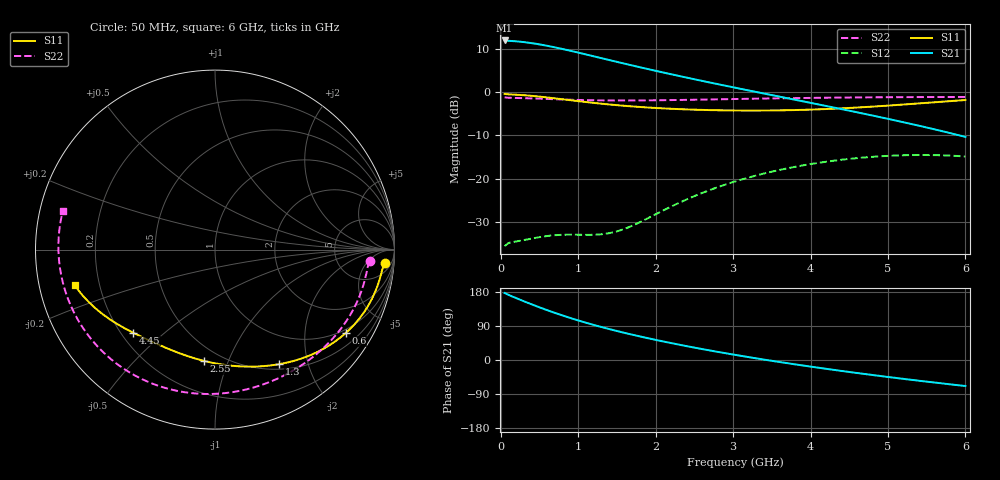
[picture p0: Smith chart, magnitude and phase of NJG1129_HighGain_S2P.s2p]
!S parameter
! Frequency  S11  S21  S12  S22
# HZ  S  DB R 50
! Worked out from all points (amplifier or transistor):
!   120 points, 50 MHz to 6 GHz, reference 50 ohm
!   highest |S21| = 11.9 dB at 50 MHz (marker M1)
!   |S21| within 3 dB of that: start of sweep to 1.047 GHz
!   unconditionally stable (mu >= 1): 116.3 MHz to 2.346 GHz
!   at 1.05 GHz: K = 1.47, MAG = 16.8 dB, |S12| = -33.0 dB
!   at 3.05 GHz: K = 0.66, MSG = 10.7 dB, |S12| = -20.5 dB
!   at 6 GHz: K = 0.66, MSG = 2.3 dB, |S12| = -14.9 dB
!   lowest NFmin = 0.69 dB at 250 MHz
!   S11 on the Smith chart (normalised r, x): 50 MHz: 12, -18; 600 MHz: 0.87, -3.21; 1.3 GHz: 0.57, -1.56; 2.55 GHz: 0.40, -0.82; 4.45 GHz: 0.25, -0.40; 6 GHz: 0.11, -0.12
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5e7  -0.45 -4.3  11.88 176.8  -35.59 29.4  -1.25 -4.3
2e8  -0.64 -11.9  11.68 163.3  -34.49 17.2  -1.39 -11.0
3.5e8  -0.82 -19.9  11.39 150.8  -34.01 20.3  -1.46 -18.5
4.5e8  -0.98 -25.1  11.13 142.9  -33.67 22.6  -1.52 -23.4
6e8  -1.27 -32.5  10.65 131.5  -33.25 25.3  -1.61 -30.6
7e8  -1.48 -37.2  10.29 124.3  -33.06 27.0  -1.68 -35.2
8e8  -1.69 -41.6  9.90 117.4  -32.96 28.8  -1.74 -39.7
9e8  -1.91 -45.8  9.50 110.8  -32.93 30.9  -1.79 -44.1
1.05e9  -2.22 -51.7  8.87 101.4  -32.96 35.3  -1.86 -50.5
1.3e9  -2.71 -60.7  7.80 87.0  -32.84 46.3  -1.94 -60.6
1.45e9  -2.97 -65.6  7.16 79.1  -32.40 54.6  -1.96 -66.4
1.65e9  -3.27 -71.8  6.32 69.1  -31.23 65.1  -1.96 -73.9
1.85e9  -3.53 -77.6  5.49 59.8  -29.59 72.8  -1.95 -81.2
2.05e9  -3.74 -83.2  4.68 51.0  -27.78 77.1  -1.91 -88.3
2.3e9  -3.96 -89.7  3.70 40.6  -25.61 78.5  -1.85 -96.8
2.55e9  -4.12 -95.9  2.74 30.8  -23.68 77.1  -1.78 -105.1
3.05e9  -4.28 -107.3  0.90 12.8  -20.53 69.4  -1.62 -120.7
3.55e9  -4.26 -117.6  -0.90 -3.7  -18.20 58.4  -1.48 -135.2
4.05e9  -4.04 -127.3  -2.69 -18.9  -16.50 45.7  -1.36 -148.7
4.45e9  -3.74 -134.7  -4.14 -30.2  -15.54 34.7  -1.29 -158.9
5.05e9  -3.09 -146.0  -6.40 -46.0  -14.71 17.3  -1.21 -173.3
6e9  -1.87 -165.8  -10.38 -68.6  -14.89 -11.5  -1.16 165.9
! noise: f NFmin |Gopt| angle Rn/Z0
5e+07  0.95  0.83  7.25  1.165
7e+08  0.768  0.673  41.14  0.381
1.35e+09  0.982  0.622  76.5  0.297
2e+09  1.244  0.578  109.1  0.199
2.65e+09  1.516  0.546  137.9  0.119
3.35e+09  1.795  0.52  163.7  0.077
4e+09  2.032  0.503  -178.3  0.08
4.65e+09  2.242  0.502  -167.4  0.102
5.3e+09  2.424  0.543  -164  0.114
6e+09  2.611  0.663  -164.3  0.108
